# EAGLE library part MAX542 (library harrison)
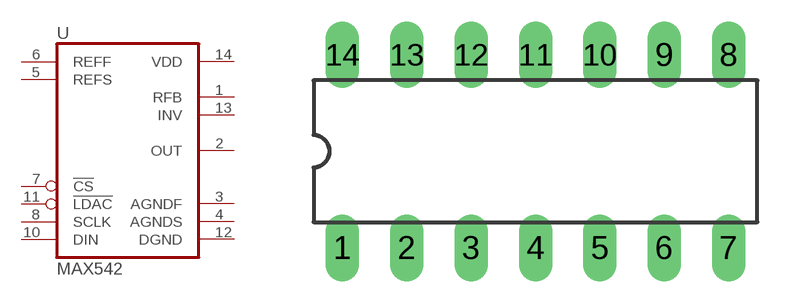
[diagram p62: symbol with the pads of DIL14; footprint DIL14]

Designator prefix U

## MAX542  [DIL14]
1  RFB  pas
2  OUT  out
3  AGNDF  pwr
4  AGNDS  pwr
5  REFS  in
6  REFF  in
7  !CS!  in
8  SCLK  in
10  DIN  in
11  !LDAC!  in
12  DGND  pwr
13  INV  pas
14  VDD  pwr

## Footprint DIL14 (pad centres in mm)
drill 0.813 long: 1 -7.62,-3.81; 2 -5.08,-3.81; 3 -2.54,-3.81; 4 0,-3.81; 5 2.54,-3.81; 6 5.08,-3.81; 7 7.62,-3.81; 8 7.62,3.81; 9 5.08,3.81; 10 2.54,3.81; 11 0,3.81; 12 -2.54,3.81; 13 -5.08,3.81; 14 -7.62,3.81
